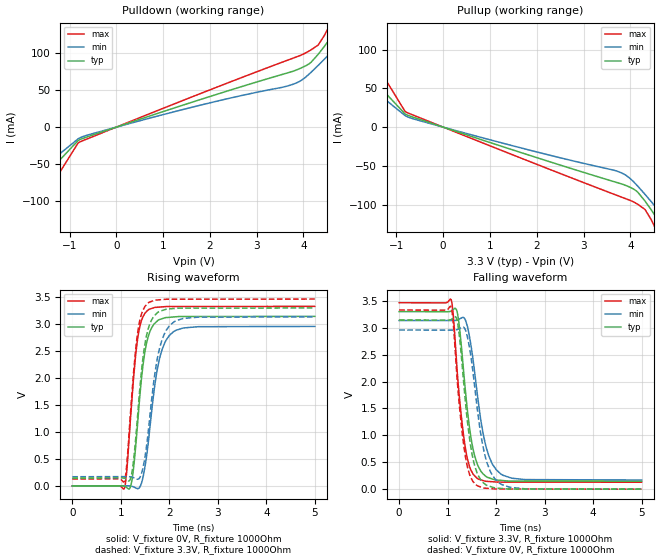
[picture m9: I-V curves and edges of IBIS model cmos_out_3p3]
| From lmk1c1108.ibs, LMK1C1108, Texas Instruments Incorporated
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[Model]   cmos_out_3p3
Model_type   Output
Polarity   Non-Inverting
Vmeas = 1.65
Vref = 0
Cref = 5pF
Rref = 100000
|   typ   min   max
C_comp   2.1615pF   1.9979pF   2.3742pF
[Voltage Range]   3.3   3.135   3.465
[Temperature Range]   25   150   -40
[Pullup Reference]   3.3   3.135   3.465
[Pulldown Reference]   -0   -0   0
[Power Clamp Reference]   3.3   3.135   3.465
[GND Clamp Reference]   0   0   0
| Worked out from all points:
|   slope of the pulldown table from 0 to 0.495 V, typ, clamps not added: 47.5 ohm
|   slope of the pullup table from 0 to 0.495 V, typ, clamps not added: 50.2 ohm
|   falling waveform, V_fixture 3.3V, R_fixture 1000Ohm: 20-80 % time 236ps typ, 297ps min, 209ps max; typ from 3.3 V to 0.147 V
|   rising waveform, V_fixture 0V, R_fixture 1000Ohm: 20-80 % time 207ps typ, 263ps min, 182ps max; typ from 0 V to 3.14 V
|   rising waveform, V_fixture 3.3V, R_fixture 1000Ohm: 20-80 % time 208ps typ, 262ps min, 185ps max; typ from 0.147 V to 3.3 V
|   falling waveform, V_fixture 0V, R_fixture 1000Ohm: 20-80 % time 230ps typ, 285ps min, 206ps max; typ from 3.14 V to 0 V
[Pulldown]
|   Voltage   I(typ)   I(min)   I(max)
-3.3V     -264.5mA   -192.3mA   -414mA
-2.874V   -209mA     -151.3mA   -327.8mA
-2.31V    -140.2mA   -105.1mA   -215.4mA
-1.904V   -98.83mA   -77.79mA   -147mA
-1.756V   -86.81mA   -68.7mA    -125.7mA
-815.1mV  -17.97mA   -15.74mA   -21.25mA
3.759V    74.97mA    57.42mA    92.52mA
4.125V    85.54mA    71.73mA    102.8mA
4.313V    98.07mA    83.14mA    110.6mA
4.531V    116.1mA    96.97mA    133.6mA
5.283V    185.3mA    145.8mA    232.9mA
6.6V      352.8mA    264.2mA    500mA
[Pullup]
|   Voltage   I(typ)   I(min)   I(max)
-3.3V     255.5mA    184.4mA    405.5mA
-2.864V   200.2mA    143.6mA    318.7mA
-2.31V    134.4mA    99.74mA    209.9mA
-1.914V   95.22mA    74.25mA    144.3mA
-1.766V   83.59mA    65.65mA    123mA
-815.1mV  17.07mA    14.95mA    20.28mA
3.759V    -72.23mA   -57.67mA   -88.99mA
4.085V    -80.45mA   -71.42mA   -96.98mA
4.313V    -95.23mA   -86.63mA   -106.1mA
4.511V    -112.4mA   -100.7mA   -127.3mA
5.283V    -186.8mA   -156.5mA   -231.7mA
6.6V      -364.2mA   -282.5mA   -504.2mA
[Ramp]
R_load = 1000
|   typ   min   max
dV/dt_r   1.88656/2.06277e-10   1.77465/2.62897e-10   1.99755/1.8207e-10
dV/dt_f   1.89161/2.35577e-10   1.77879/2.96776e-10   2.00166/2.08522e-10
[Falling Waveform]
V_fixture = 3.3V
V_fixture_min = 3.135V
V_fixture_max = 3.465V
R_fixture = 1000Ohm
C_fixture = 0F
|   Time   V(typ)   V(min)   V(max)
0s        3.3V       3.135V     3.465V
1.069ns   3.307V     3.133V     3.527V
1.117ns   3.339V     3.133V     3.222V
1.203ns   3.265V     3.144V     2.122V
1.354ns   1.946V     3.165V     833mV
1.473ns   1.005V     2.716V     368.4mV
1.604ns   484.5mV    1.821V     204.4mV
1.804ns   229.4mV    748.9mV    145.5mV
2.143ns   159.8mV    257.7mV    131.3mV
5ns       147.3mV    170.3mV    128.9mV
[Rising Waveform]
V_fixture = 0V
V_fixture_min = 0V
V_fixture_max = 0V
R_fixture = 1000Ohm
C_fixture = 0F
|   Time   V(typ)   V(min)   V(max)
0s        15.23uV    14.75uV    16.26uV
1.074ns   -4.969mV   2.362mV    -46.48mV
1.126ns   -32.61mV   2.476mV    302mV
1.224ns   72.86mV    -6.456mV   1.534V
1.339ns   1.068V     -49.6mV    2.671V
1.457ns   2.23V      156.1mV    3.136V
1.559ns   2.748V     744.2mV    3.259V
1.789ns   3.081V     2.32V      3.316V
2.093ns   3.133V     2.863V     3.327V
5ns       3.144V     2.958V     3.329V
[Rising Waveform]
V_fixture = 3.3V
V_fixture_min = 3.135V
V_fixture_max = 3.465V
R_fixture = 1000Ohm
C_fixture = 0F
|   Time   V(typ)   V(min)   V(max)
0s        147.3mV    170.3mV    128.9mV
1.074ns   142.5mV    172.5mV    83.56mV
1.126ns   116.2mV    172.6mV    420.3mV
1.224ns   219.6mV    164.9mV    1.64V
1.339ns   1.216V     124.1mV    2.78V
1.457ns   2.372V     335mV      3.259V
1.559ns   2.891V     946.8mV    3.39V
1.789ns   3.233V     2.512V     3.45V
2.093ns   3.289V     3.04V      3.462V
5ns       3.3V       3.135V     3.465V
[Falling Waveform]
|Gnd
V_fixture = 0V
V_fixture_min = 0V
V_fixture_max = 0V
R_fixture = 1000Ohm
C_fixture = 0F
|   Time   V(typ)   V(min)   V(max)
0s        3.144V     2.958V     3.329V
1.069ns   3.151V     2.956V     3.391V
1.117ns   3.186V     2.956V     3.071V
1.203ns   3.102V     2.967V     1.962V
1.339ns   1.893V     3.002V     771.1mV
1.457ns   908.5mV    2.595V     260.6mV
1.588ns   352mV      1.665V     79mV
1.817ns   67.01mV    475.2mV    15.34mV
2.12ns    12.66mV    84.63mV    3.174mV
5ns       15.23uV    14.75uV    16.26uV
